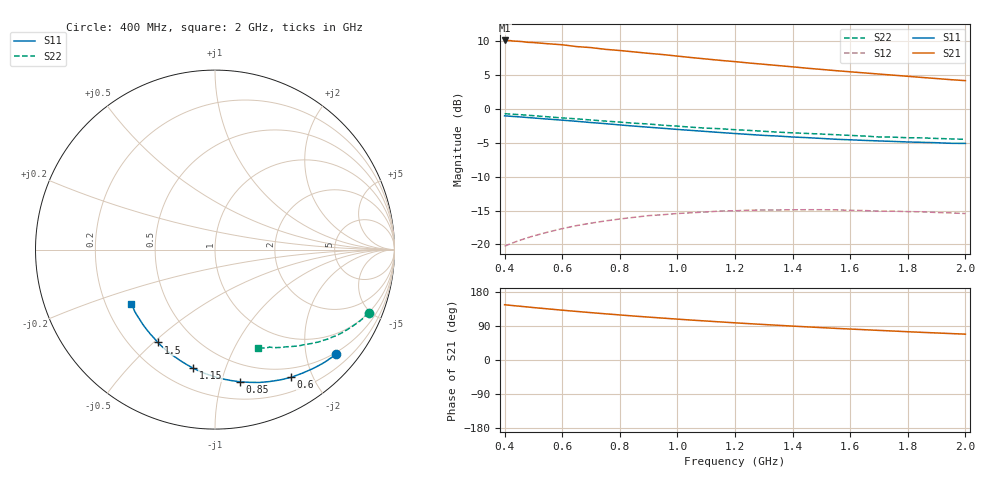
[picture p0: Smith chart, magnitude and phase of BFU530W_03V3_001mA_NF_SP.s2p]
! Filename:  P:\Prog\Test\Noise\ATS_data\Testdata_Net\06 Compressed Noise after Statistics\BFU530W_APM2013_09_A05_03p3V_001mA_NF_CM01_D.sf
! Date/Time: Tue 26/Mar/2013 18:06:08
! BFU530W_APM2013_09_A05_03p3V_1to25mA_NF_CM01_Bias1_R.sf
! Noise Parameter Data File
! BFU530W_APM2013_09_A05_03p3V_1to25mA_NF_CM01
! Date/time: Thu Mar 21 19:18:02 2013
! freq range =  0.4000 to  2.0000 GHz, 37 points
! bias range =  0.9950 to 25.0000 mA, 9 points
! bias supplies used: 1 1 0 0 0 0
! VAR bias_mode= 1  ! Specify V_out, I_out
! VAR bias_var = 1  ! Bias variable = I_out
! VAR V_out= 3.300000
! VAR I_out= 0.995000
! VAR V_in= 0.783400
! VAR I_in= 0.010301
! Device data file deembeded for feedlines and parallel
! Original file: \06 Compressed Noise after Statistics\BFU530W_APM2013_09_A05_03p3V_001mA_NF_CM01_R.sf
! Feed-files: PR019V01_070313_Feed1.s2p, PR019V01_070313_Feed2.s2p
! Parallel-file: PR019V01_070313_Par.s2p
# MHz S MA R 50
!  Freq-MHz  S11-mag  S11-arg  S21-mag  S21-arg  S12-mag  S12-arg  S22-mag  S22-arg
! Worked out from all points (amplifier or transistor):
!   37 points, 400 MHz to 2 GHz, reference 50 ohm
!   highest |S21| = 10.1 dB at 400 MHz (marker M1)
!   |S21| within 3 dB of that: start of sweep to 1.165 GHz
!   unconditionally stable (mu >= 1): nowhere
!   at 500 MHz: K = 0.20, MSG = 14.3 dB, |S12| = -18.7 dB
!   at 1.1 GHz: K = 0.41, MSG = 11.3 dB, |S12| = -15.2 dB
!   at 2 GHz: K = 0.75, MSG = 9.8 dB, |S12| = -15.4 dB
!   lowest NFmin = 0.44 dB at 420 MHz
!   S11 on the Smith chart (normalised r, x): 400 MHz: 0.46, -2.62; 600 MHz: 0.37, -1.70; 850 MHz: 0.34, -1.15; 1.15 GHz: 0.32, -0.78; 1.5 GHz: 0.31, -0.52; 2 GHz: 0.31, -0.27
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400  0.8921 -40.7  3.215 145.9  0.09717 64.1  0.9248 -22.3
420  0.8856 -42.7  3.205 144.3  0.1012 62.9  0.919 -23.3
433  0.8811 -43.8  3.18 143.3  0.1037 62.2  0.9153 -23.9
460  0.8734 -46.5  3.154 141.4  0.1086 60.7  0.9075 -25.1
480  0.8667 -48.2  3.115 139.9  0.1122 59.6  0.9013 -26.1
500  0.8599 -50.2  3.102 138.4  0.1156 58.6  0.8941 -26.9
600  0.8287 -59.1  2.988 131.5  0.1309 53.7  0.8611 -31.2
650  0.8126 -63.2  2.896 128.2  0.1379 51.5  0.8474 -33.0
700  0.7955 -67.5  2.847 125.0  0.1437 49.2  0.8307 -35.1
750  0.7807 -71.5  2.764 121.9  0.1493 47.3  0.8155 -36.7
800  0.7641 -75.5  2.709 118.9  0.1543 45.3  0.8017 -38.5
850  0.749 -79.4  2.646 115.9  0.1588 43.5  0.7866 -40.0
950  0.7215 -86.8  2.527 110.5  0.166 40.0  0.7599 -43.1
1050  0.6955 -93.8  2.401 105.3  0.1716 37.1  0.735 -45.8
1150  0.6714 -100.5  2.29 100.4  0.1767 34.3  0.7163 -48.2
1200  0.6601 -103.7  2.242 98.1  0.1774 33.1  0.7043 -49.7
1350  0.6321 -112.9  2.097 91.6  0.18 29.9  0.6759 -53.2
1500  0.6073 -121.6  1.964 85.4  0.1806 27.2  0.6541 -56.5
1600  0.5932 -127.2  1.886 81.7  0.1789 25.8  0.6395 -58.7
1750  0.5771 -134.9  1.781 76.4  0.1763 24.6  0.6207 -61.5
1850  0.5683 -139.9  1.713 72.9  0.1742 23.8  0.6128 -63.5
2000  0.5577 -147.2  1.623 68.2  0.1693 23.7  0.5981 -66.5
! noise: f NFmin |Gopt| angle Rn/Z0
400  0.4503  0.6776  25.09  0.309
460  0.4909  0.6646  29.66  0.327
600  0.5215  0.676  37.29  0.3245
800  0.6505  0.6112  50.98  0.2748
1000  0.754  0.6381  62.28  0.2989
1200  0.7626  0.6184  75.19  0.2535
1400  0.8184  0.5868  87.29  0.2086
1600  0.7679  0.5611  99.96  0.15
1800  0.9911  0.5164  113.9  0.1543
2000  1.1  0.5271  125.9  0.1298
